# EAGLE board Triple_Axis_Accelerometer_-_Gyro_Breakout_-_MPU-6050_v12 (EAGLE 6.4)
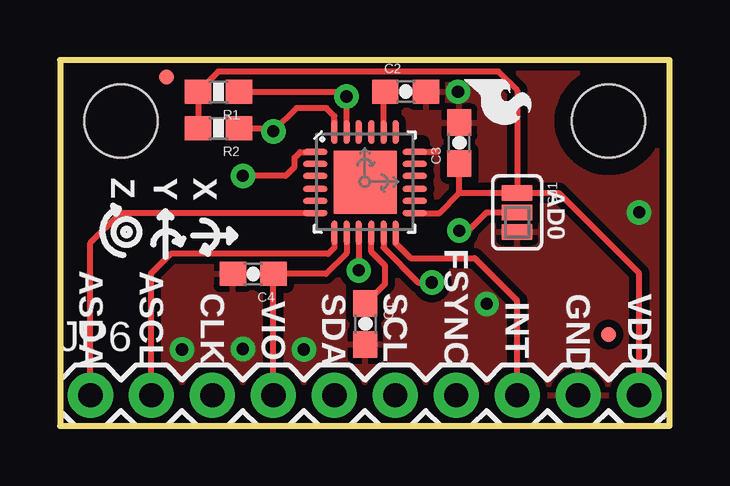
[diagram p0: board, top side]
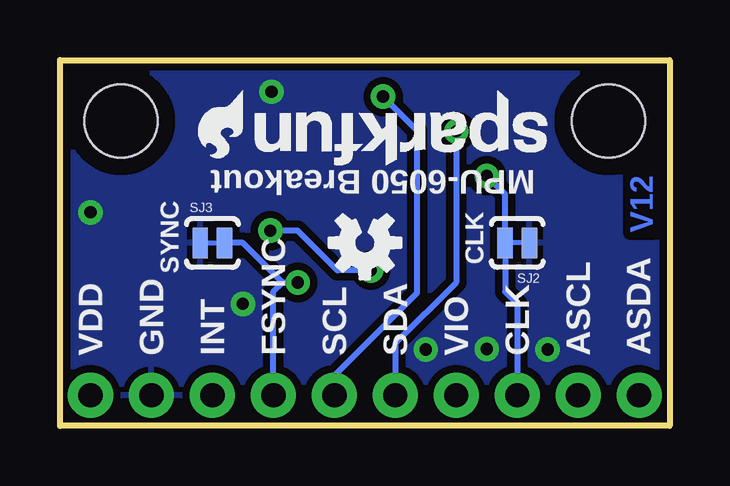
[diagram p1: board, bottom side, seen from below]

Size 25.4 x 15.24 mm. Coordinates in mm from the lower left corner, seen from the top.
Outline: 25.4,0 25.4,15.24 0,15.24 0,0 25.4,0
Copper layers (1*16): Top 0.035mm / dielectric 1.5mm / Bottom 0.035mm
Design rules "SparkFun *": minimum track width 7mil, minimum drill 15mil, track to track 8mil, track to pad 8mil, pad to pad 8mil, via to via 8mil, smd to smd 8mil, copper to edge 8mil, drill to drill 8mil, minimum pad ring 12mil, minimum via ring 10mil, stop-mask expansion 4mil, vias tented up to drill 20mil, thermal gap 10mil
Net classes: 0 Default: width 0.203 mm; 1 vcc: width 0.254 mm; 2 GND: width 0.813 mm
tRestrict: area 14.5,11.6 to 15.1,11.8

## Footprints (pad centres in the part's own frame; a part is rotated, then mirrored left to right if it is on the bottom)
0603-CAP = smd 1.1 x 1: 1 -0.85,0; 2 0.85,0
MICRO-FIDUCIAL = smd 0.635 x 0.635: 1 0,0
STAND-OFF-TIGHT = hole 3.048: 0,0
1X10 = drill 1.016 pad 1.88: 1 0,0; 2 2.54,0; 3 5.08,0; 4 7.62,0; 5 10.16,0; 6 12.7,0; 7 15.24,0; 8 17.78,0; 9 20.32,0; 10 22.86,0
0603-RES = smd 1.1 x 1: 1 -0.85,0; 2 0.85,0
SJ_3_PASTE2&3 = smd 0.635 x 1.27: 1 -0.813,0; 2 0,0; 3 0.813,0
SJ_2S-TRACE = smd 0.635 x 1.27: 1 -0.508,0; 2 0.508,0
QFN-24-4MM2 = smd 1.016 x 0.254: 1 -2.066,1.257; 2 -2.066,0.75; 3 -2.066,0.247; 4 -2.066,-0.287; 5 -2.066,-0.792; 6 -2.066,-1.297; 13 2.086,-1.297; 14 2.086,-0.792; 15 2.086,-0.287; 16 2.086,0.247; 17 2.086,0.75; 18 2.086,1.257 | smd 0.254 x 1.016: 7 -1.267,-2.122; 8 -0.762,-2.122; 9 -0.258,-2.122; 10 0.278,-2.122; 11 0.78,-2.122; 12 1.287,-2.122; 19 1.287,2.082; 20 0.78,2.082; 21 0.278,2.082; 22 -0.258,2.082; 23 -0.762,2.082; 24 -1.267,2.082 | smd 2.616 x 2.616: P$1 0.02,-0.01

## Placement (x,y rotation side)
C1  0.1uF  [0603-CAP]  12.73,4.24 270 top
C2  2.2nF  [0603-CAP]  14.4,13.92 0 top
C3  0.1uF  [0603-CAP]  16.64,11.79 90 top
C4  10nF  [0603-CAP]  8.05,6.32 180 top
FRAME1  FRAME-LETTER  [CREATIVE_COMMONS]  not placed on the board
JP2  FIDUCIALUFIDUCIAL  [MICRO-FIDUCIAL]  4.45,14.53 270 top
JP3  STAND-OFFTIGHT  [STAND-OFF-TIGHT]  22.86,12.7 270 top
JP4  STAND-OFFTIGHT  [STAND-OFF-TIGHT]  2.54,12.7 270 top
JP5  FIDUCIALUFIDUCIAL  [MICRO-FIDUCIAL]  22.86,3.81 270 top
JP6  M10"  [1X10]  1.27,1.27 0 top
R1  10k  [0603-RES]  6.6,13.92 180 top
R2  10k  [0603-RES]  6.6,12.4 180 top
SJ1  [SJ_3_PASTE2&3]  19.05,8.89 270 top
SJ2  [SJ_2S-TRACE]  6.35,7.62 180 bottom
SJ3  [SJ_2S-TRACE]  19.05,7.62 0 bottom
U1  MPU-6050-1  [QFN-24-4MM2]  12.7,10.16 0 top
U$1  OSHW-LOGOS  [OSHW-LOGO-S]  12.7,7.62 180 bottom
U$2  [SFE-LOGO-FLAME]  16.84,14.43 270 top
U$3  [SFE-LOGO-FLAME]  17.78,13.97 180 bottom
U$4  [SFE-NEW-WEB]  5.08,13.97 180 bottom
U$5  REVISION  [REVISION]  not placed on the board

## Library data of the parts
C1-C4 JP2-JP6 R1 R2 SJ1-SJ3 U$1-U$4 = SparkFun
FRAME1 U$5 = SparkFun-Aesthetics
U1 = Testing

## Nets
ADO: SJ1.2 U1.9
AUX_SCL: JP6.2 U1.7
AUX_SDA: JP6.1 U1.6
CLKIN: JP6.3 SJ2.2 U1.1
FSYNC: JP6.7 SJ3.2 U1.11
GND: C1.2 C2.2 C3.2 C4.2 JP6.9 SJ1.3 SJ2.1 SJ3.1 U1.18
INT: JP6.8 U1.12
N$3: C2.1 U1.20
N$5: C1.1 U1.10
SCL: JP6.6 R1.1 U1.23
SDA: JP6.5 R2.1 U1.24
VCC: C3.1 JP6.10 R1.2 R2.2 SJ1.1 U1.13
VIO: C4.1 JP6.4 U1.8

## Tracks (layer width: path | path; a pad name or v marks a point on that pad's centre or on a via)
ADO  (via drill 0.51)
  Top 0.254: v16.64,8.13 17.02,8.13 17.78,8.89 SJ1.2 | U1.9 v12.44,6.48 v12.45,6.48
  Bottom 0.254: v12.45,6.48 13.84,6.48 15.49,8.13 v16.64,8.13
AUX_SCL
  Top 0.254: U1.7 11.43,7.42 11.18,7.16 4.62,7.16 3.79,6.33 3.79,1.29 JP6.2
AUX_SDA
  Top 0.254: JP6.1 1.27,7.62 2.51,8.86 U1.6
CLKIN  (via drill 0.51)
  Top 0.254: v7.62,10.41 9.4,10.41 9.78,10.79 9.78,11.18 10.01,11.4 10.62,11.4 U1.1
  Bottom 0.254: v7.62,10.41 6.86,9.65 SJ2.2 6.86,5.59 6.35,5.08 JP6.3
FSYNC  (via drill 0.51)
  Top 0.254: U1.11 13.48,7.42 14.94,5.97 v15.49,5.97
  Bottom 0.254: JP6.7 16.51,5.59 16.13,5.97 | v15.49,5.97 16.13,5.97 | 16.13,5.97 17.78,7.62 SJ3.2
GND  (via drill 0.51)
  Top 0.254: U1.18 15.66,11.42 15.67,11.43
  other vias: 16.59,13.92 17.78,5.08 24.13,8.89 10.16,3.17 7.62,3.2 5.08,3.17
  pour Top (isolate 0.305): 25.4,15.24 0,15.24 0,0 25.4,0
  pour Bottom (isolate 0.305): 25.4,15.24 0,15.24 0,0 25.4,0
INT
  Top 0.254: JP6.8 19.05,5.21 17.27,6.99 14.61,6.99 13.99,7.6 U1.12
N$3
  Top 0.254: U1.20 13.48,13.92 C2.1
N$5
  Top 0.254: C1.1 13.54,5.91 13.54,6.68 12.98,7.24 U1.10
SCL  (via drill 0.51)
  Top 0.254: U1.23 v11.94,13.72 | v11.94,13.72 | R1.1 11.73,13.92 v11.94,13.72
  Bottom 0.254: v11.94,13.72 10.52,12.29 10.52,5.54 13.97,2.08 JP6.6
SDA  (via drill 0.51)
  Top 0.254: U1.24 11.43,12.7 | 11.43,12.72 11.43,12.7 | 11.43,12.7 11.43,12.9 11.1,13.23 9.86,13.23 v8.89,12.27 | 8.87,12.24 v8.89,12.27 | R2.1 8.76,12.39 v8.89,12.27
  Bottom 0.254: v8.89,12.27 8.89,5.97 11.43,3.43 JP6.5
VCC
  Top 0.254: SJ1.1 20.78,9.7 24.13,6.35 JP6.10 | R2.2 R1.2 6.59,14.76 18.26,14.76 19.05,13.97 SJ1.1 | 16.36,10.66 C3.1 16.64,9.7 | U1.13 15.8,8.86 16.64,9.7 | 16.64,9.7 SJ1.1
VIO
  Top 0.254: JP6.4 C4.1 | 8.93,6.35 C4.1 | 9.11,6.53 C4.1 | U1.8 11.94,7.19 11.07,6.33 C4.1

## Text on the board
Bottom: V12
tPlace: Z | Y | X | AD0 | FSYNC | ASDA | ASCL | CLK | SDA | SCL | GND | VDD | VIO | INT
bPlace: MPU-6050 Breakout | CLK | SYNC | ASDA | ASCL | CLK | VIO | SDA | SCL | FSYNC | INT | GND | VDD
tValues: Joel Bartlett | Eric Orosel

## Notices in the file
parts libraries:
SparkFun-Aesthetics: Licensing: CC v3.0 Share-Alike You are welcome to use this library for commercial purposes.
SparkFun-Aesthetics: Released under the Creative Commons Attribution Share-Alike 3.0 License
SparkFun-Aesthetics: http://creativecommons.org/licenses/by-sa/3.0
